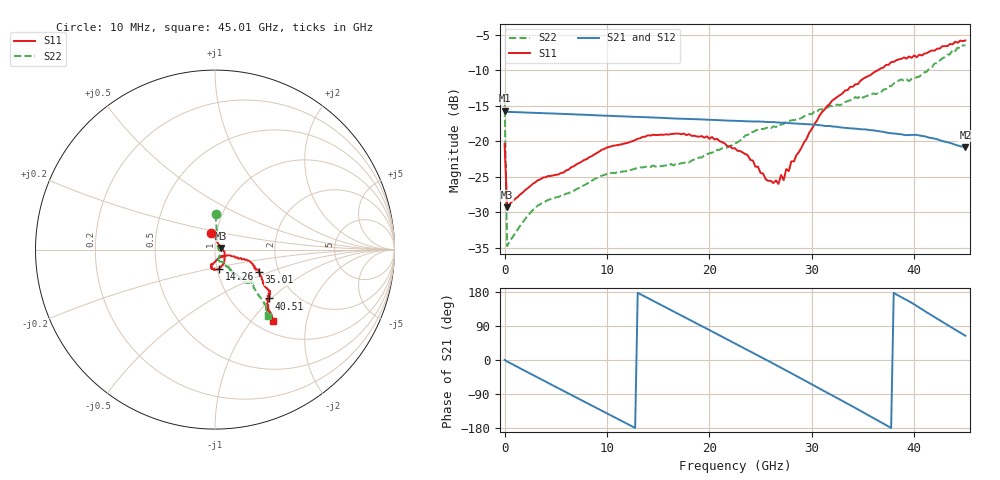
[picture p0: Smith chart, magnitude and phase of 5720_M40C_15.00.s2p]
! Device:  ADRF5720
! Description: 0.5dB LSB GaAs MMIC 6-bit Digital Attenuator
! Frequency:  0.000009 -  40 GHz
! Ports:
!	RF1	= Port 1
!	RF2	= Port 2
! Vdd:  3.3 Volt
! Vss:  -3.3 Volt
! Control:  0/3.3 Volt
! State:  15.00 dB attenuation
! Data:  The device was measured using G-S-G Probes on a matrix board.
!  Data was collected using an calibrated 4 port network analyzer.
!  The reference plane for this measurement is at the launchers.
! Note:  Analog Devices supplies this data as a sample of measured data
!  for this product.  Your particular data for this product may vary.
!  Data was taken at -40 degrees C.
!  Analog Devices reserves the right to change this data at anytime.
# GHZ S DB R 45.0
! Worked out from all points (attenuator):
!   181 points, 10 MHz to 45.01 GHz, reference 45 ohm
!   highest |S21| = -15.70 dB at 10 MHz (marker M1); lowest = -20.9 dB at 45.01 GHz (marker M2)
!   lowest |S11| = -29.4 dB at 260 MHz (marker M3), VSWR 1.07, Z = 48.1 + j0.843 ohm
!   |S11| at or under -10 dB: start of sweep to 36.48 GHz
!   |S22| runs from -34.8 to -6.5 dB; largest |S21 - S12| = 0.00062
!   S11 on the Smith chart (normalised r, x): 10 MHz: 0.94, +0.18; 14.26 GHz: 1.02, -0.22; 35.01 GHz: 1.58, -0.43; 40.51 GHz: 1.49, -0.97; 45.01 GHz: 1.19, -1.29
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0.01  -20.39 102.2  -15.70 0.2  -15.72 0.2  -14.10 89.2
0.26  -29.36 14.9  -15.88 -3.9  -15.89 -3.9  -34.81 25.8
3.26  -25.52 -12.8  -16.04 -46.5  -16.07 -46.5  -29.07 -30.6
7.76  -22.68 -43.4  -16.29 -109.5  -16.31 -109.5  -26.22 -64.6
11.26  -20.51 -61.3  -16.50 -158.3  -16.52 -158.4  -24.41 -74.2
14.26  -19.22 -77.7  -16.67 159.7  -16.68 159.6  -23.63 -76.1
15.26  -19.09 -82.1  -16.72 145.6  -16.74 145.5  -23.55 -75.0
20.26  -19.42 -100.0  -17.01 75.4  -17.03 75.3  -21.62 -58.9
22.76  -21.37 -104.7  -17.16 40.2  -17.18 40.1  -20.17 -56.7
23.76  -22.01 -99.3  -17.22 26.1  -17.25 26.0  -19.15 -56.1
25.51  -25.40 -75.2  -17.30 1.0  -17.32 0.9  -18.19 -53.0
26.76  -26.04 -50.0  -17.39 -16.9  -17.42 -17.1  -17.69 -51.9
27.01  -24.78 -45.4  -17.41 -20.4  -17.43 -20.6  -17.70 -53.4
27.26  -25.51 -42.1  -17.41 -24.1  -17.43 -24.2  -17.57 -51.7
27.51  -23.95 -36.4  -17.41 -27.7  -17.43 -27.9  -17.36 -52.9
27.76  -24.22 -32.9  -17.47 -31.4  -17.50 -31.6  -17.19 -51.3
30.26  -17.64 -18.9  -17.69 -67.9  -17.71 -68.0  -15.85 -52.5
32.01  -14.28 -18.5  -17.94 -93.5  -17.96 -93.7  -15.06 -50.0
35.01  -11.23 -27.1  -18.35 -137.6  -18.38 -137.7  -13.89 -48.6
37.76  -8.87 -36.9  -18.90 -179.4  -18.92 -179.6  -12.25 -48.1
40.51  -7.83 -42.1  -19.21 138.1  -19.24 137.9  -10.91 -43.6
45.01  -5.82 -51.0  -20.87 64.0  -20.90 63.9  -6.49 -51.5
